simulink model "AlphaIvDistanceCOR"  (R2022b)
settings: Solver=FixedStepAuto  StartTime=0.0  StopTime=20/40000  FixedStep=1/4000000000  RelTol=1e-3

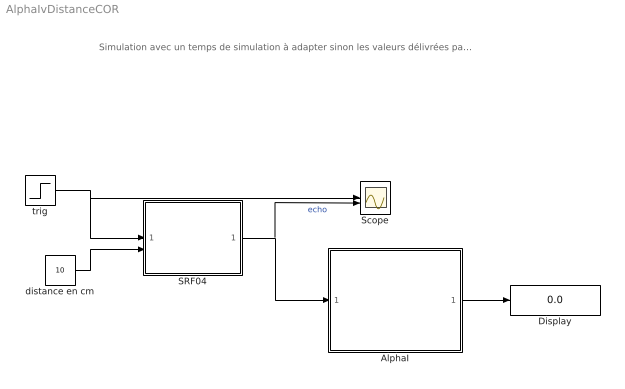
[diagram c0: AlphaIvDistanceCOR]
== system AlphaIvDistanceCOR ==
  note: Simulation avec un temps de simulation à adapter sinon les valeurs délivrées par le capteur vont se figer : idéal à 20/40000 On peut amélioer la "justesse" du capteur en dimiunuant le Fixe step Size 1/40 000 000, dans l'onglet modeling puis modeling setting
  AlphaI : Subsystem
  Display : Display
  SRF04 : Subsystem
  Scope : Scope  NumInputPorts=2
  distance en cm : Constant  Value=10
  trig : Step  Time=6/400000  Before=1  After=0  SampleTime=0
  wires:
  trig/1 -> Scope/1, SRF04/1(Trig)
  SRF04/1(echo) -> AlphaI/1(echo), Scope/2  "echo"
  distance en cm/1 -> SRF04/2(distance)
  AlphaI/1(distance) -> Display/1

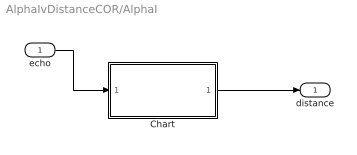
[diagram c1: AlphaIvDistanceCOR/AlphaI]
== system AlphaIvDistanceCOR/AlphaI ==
  echo : Inport
  Chart : Stateflow chart  TreatAsAtomicUnit=on
  distance : Outport
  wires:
  Chart/1(distance) -> distance/1
  echo/1 -> Chart/1(echo)

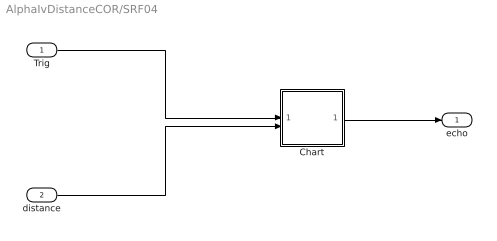
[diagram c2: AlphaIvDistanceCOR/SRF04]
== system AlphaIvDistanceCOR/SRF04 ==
  Trig : Inport
  distance : Inport  Port=2
  Chart : Stateflow chart  TreatAsAtomicUnit=on
  echo : Outport  VectorParamsAs1DForOutWhenUnconnected=off
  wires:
  Trig/1 -> Chart/1(trig)
  distance/1 -> Chart/2(d)
  Chart/1(echo) -> echo/1

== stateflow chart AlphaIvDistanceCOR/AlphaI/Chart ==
  state attente
    cpt=0;
  state affichage
  state comptage
    entry:
    cpt=cpt+1
    exit:
    distance=cpt/10
  (default) -> attente
  attente -> affichage : [echo]
  comptage -> affichage : [echo==1]
  affichage -> comptage : after(0.17,usec)
  comptage -> (junction 10) : [echo==0]
  data: echo input; distance output; cpt local

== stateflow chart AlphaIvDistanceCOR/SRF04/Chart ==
  state attente
    echo=0;
  state attente1
  state echo
    echo=1;
  (default) -> attente
  echo -> attente : after(0.0001*d/58,sec)
  attente -> attente1 : [trig==1]
  attente1 -> echo : after(0.0001,sec)
  data: trig input; d input; echo output
